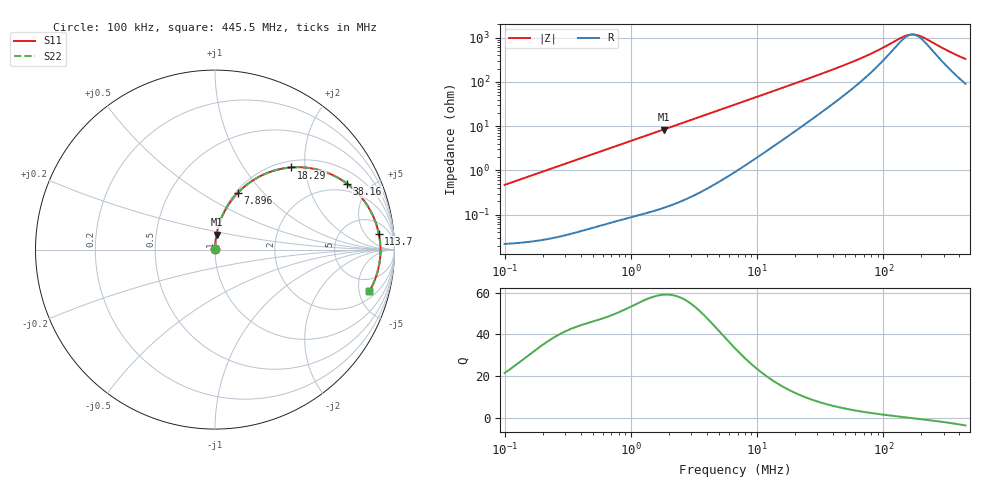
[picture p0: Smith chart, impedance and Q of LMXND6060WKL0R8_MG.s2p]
! LMXND6060WKL0R8_MG  S-PARAMETER MODEL  ( General Type )
! Model Generated by TAIYO YUDEN Corporation (http://www.ty-top.com)
! Version 1.0
! TAIYO YUDEN Control No. 191025NI43SB-FBB
! Copyright(c) 2019 TAIYO YUDEN CO.,LTD. All Rights Reserved.
! Product Description (link to TY-COMPAS)
! https://ds.yuden.co.jp/TYCOMPAS/or/detail?pn=LMXND6060WKL0R8NMG&u=M
! Products Name : Inductors
! Characteristics :
!  Inductance : 0.80 uH , SRF(min) : 110 MHz , DC Resistance(max) : 0.024 Ohm
!  Rated Current : Saturation :6400 mA , Temp Rise : 4100 mA
!  Case Size : 6.0 x 6.0 / 0.236 x 0.236 [mm/inch] , Thickness : 2 / 0.079 [mm/inch]
!  (Conditions: Temperature = 25 degC , DC Bias Current/Voltage = 0A / 0V)
! External Node Assignments :
!  1  o---GGG---o  2
! GND o---------o GND
! Frequency Range : 0.1MHz  -  445.549718MHz  [ 402 STEP ]
# MHz S RI R 50
! Freq[MHz].  S11 Real  S11 Imag  S21 Real  S21 Imag  S12 Real  S12 Imag  S22 Real  S22 Imag
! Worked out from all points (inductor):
!   401 points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, 100 kHz to 445.5 MHz, reference 50 ohm
!   read as one part in series: L = 749 nH near 104.3 kHz
!   highest Q = 59 at 1.815 MHz (marker M1), where L = 735 nH
!   self-resonance near 169.7 MHz
!   S11 on the Smith chart (normalised r, x): 100 kHz: 1.00, +0.01; 7.896 MHz: 1.03, +0.73; 18.29 MHz: 1.13, +1.69; 38.16 MHz: 1.58, +3.60; 113.7 MHz: 10, +11; 445.5 MHz: 2.82, -6.34
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0.1  0.00024 0.00471  0.9998 -0.00471  0.9998 -0.00471  0.00024 0.00471
0.408498  0.000794 0.0191  0.9992 -0.0191  0.9992 -0.0191  0.000794 0.0191
1.668708  0.00719 0.0764  0.9928 -0.0764  0.9928 -0.0764  0.00719 0.0764
1.814969  0.00836 0.083  0.9916 -0.083  0.9916 -0.083  0.00836 0.083
3.554519  0.0291 0.1586  0.9709 -0.1586  0.9709 -0.1586  0.0291 0.1586
6.81664  0.097 0.2811  0.903 -0.2811  0.903 -0.2811  0.097 0.2811
7.896343  0.1255 0.3145  0.8745 -0.3145  0.8745 -0.3145  0.1255 0.3145
11.76924  0.2392 0.4026  0.7608 -0.4026  0.7608 -0.4026  0.2392 0.4026
18.29429  0.425 0.4578  0.575 -0.4578  0.575 -0.4578  0.425 0.4578
27.26705  0.609 0.4344  0.391 -0.4344  0.391 -0.4344  0.609 0.4344
38.15874  0.7369 0.3666  0.2631 -0.3666  0.2631 -0.3666  0.7369 0.3666
50.13987  0.8118 0.2959  0.1882 -0.2959  0.1882 -0.2959  0.8118 0.2959
68.7095  0.8684 0.2121  0.1316 -0.2121  0.1316 -0.2121  0.8684 0.2121
88.40639  0.896 0.1486  0.104 -0.1486  0.104 -0.1486  0.896 0.1486
111.3854  0.9114 0.0939  0.0886 -0.0939  0.0886 -0.0939  0.9114 0.0939
113.7498  0.9124 0.0891  0.0876 -0.0891  0.0876 -0.0891  0.9124 0.0891
149.4651  0.9208 0.0279  0.0792 -0.0279  0.0792 -0.0279  0.9208 0.0279
166.0164  0.9218 0.00481  0.0782 -0.00481  0.0782 -0.00481  0.9218 0.00481
180.5676  0.9218 -0.0137  0.0782 0.0137  0.0782 0.0137  0.9218 -0.0137
204.8204  0.9203 -0.0416  0.0797 0.0416  0.0797 0.0416  0.9203 -0.0416
325.1341  0.8976 -0.1499  0.1024 0.1499  0.1024 0.1499  0.8976 -0.1499
445.5497  0.8605 -0.2316  0.1395 0.2316  0.1395 0.2316  0.8605 -0.2316
